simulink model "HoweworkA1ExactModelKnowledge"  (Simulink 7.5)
settings: Solver=ode45  StartTime=0.0  StopTime=10.0  RelTol=1e-3

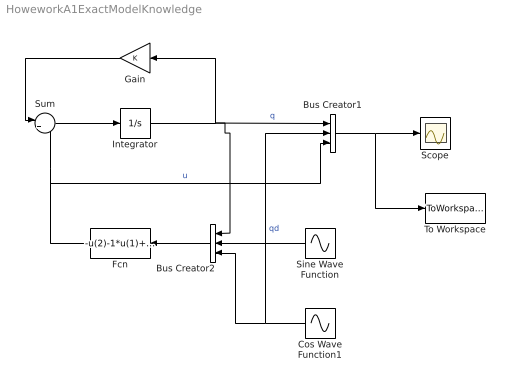
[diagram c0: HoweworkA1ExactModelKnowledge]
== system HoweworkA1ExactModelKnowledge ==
  Bus Creator1 : BusCreator  Inputs=3
  Bus Creator2 : BusCreator  Inputs=3
  Cos Wave Function1 : Sin  Amplitude=1  Bias=0  Frequency=1  Phase=pi/2  Samples=10  SampleTime=0
  Fcn : Fcn  Expr=-u(2)-1*u(1)+10*(u(3)-u(1))
  Gain : Gain  ParameterDataType=fixdt(1, 16)  ParameterScaling=2^0  OutDataType=fixdt(1, 16)  OutScaling=2^0
  Integrator : Integrator
  Scope : Scope
  Sine Wave Function : Sin  Amplitude=1  Bias=0  Frequency=1  Phase=0  Samples=10  SampleTime=0
  Sum : Sum  Inputs=|++  OutDataType=fixdt(1, 16)  OutScaling=2^0
  To Workspace : ToWorkspace  VariableName=ICP  SampleTime=-1  SaveFormat=Structure With Time
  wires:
  Integrator/1 -> Gain/1, Bus Creator1/1, Bus Creator2/1  "q"
  Sum/1 -> Integrator/1
  Gain/1 -> Sum/1
  Bus Creator1/1 -> Scope/1, To Workspace/1
  Fcn/1 -> Sum/2, Bus Creator1/3  "u"
  Bus Creator2/1 -> Fcn/1
  Cos Wave Function1/1 -> Bus Creator2/3, Bus Creator1/2  "qd"
  Sine Wave Function/1 -> Bus Creator2/2
